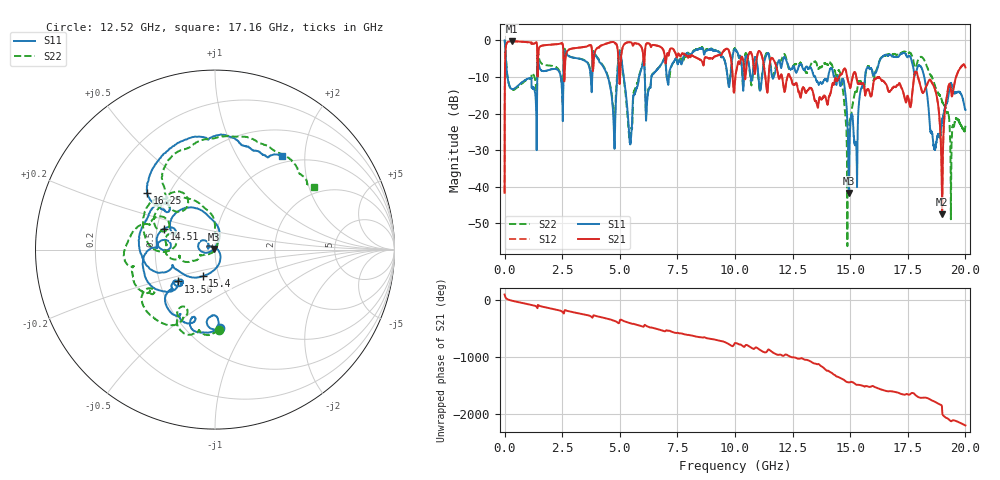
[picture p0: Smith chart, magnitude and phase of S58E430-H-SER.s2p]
!{S58E430}
!Johanson Technology Inc.
!www.johansontechnology.com
!Test Board Conditions:
!Substrate Type  RO4350B
!Substrate Thickness  60 mil
!Substrate Dk  3.66
!TL Type: GCPW
!TL Trace Width  115 mil
!TL Gap  52 mil
!Electrode orientation  Horizontal
!DUT TOPOLOGY	SERIES
!Mounting Pad LxW  55x428 mil
! Created Wed Apr 14 11:48:31 2021
# mhz S ma R 50
! 2 Port Network Data from SP1.SP block
! freq  magS11  angS11  magS21  angS21  magS12  angS12  magS22  angS22
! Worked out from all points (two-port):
!   20001 points, 300 kHz to 20 GHz, reference 50 ohm
!   highest |S21| = -0.24 dB at 309.3 MHz (marker M1); lowest = -47.5 dB at 18.99 GHz (marker M2)
!   |S21| within 3 dB of the highest: 35.1 MHz to 1.418 GHz (1.383 GHz wide, 190 % of centre); 2.697 GHz to 3.796 GHz (1.099 GHz wide, 33.8 % of centre)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
!   lowest |S11| = -41.6 dB at 14.94 GHz (marker M3), VSWR 1.02, Z = 49.3 + j0.339 ohm
!   |S11| at or under -10 dB: 125.9 MHz to 1.416 GHz (1.29 GHz wide, 167 % of centre); 14.5 GHz to 15.65 GHz (1.149 GHz wide, 7.62 % of centre); 18.21 GHz to end of sweep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
!   |S22| runs from -56.2 to 0.0 dB; largest |S21 - S12| = 0.01
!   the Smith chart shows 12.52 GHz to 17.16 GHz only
!   S11 on the Smith chart (normalised r, x): 12.52 GHz: 0.72, -0.77; 13.56 GHz: 0.62, -0.24; 14.51 GHz: 0.54, +0.14; 15.4 GHz: 0.84, -0.25; 16.25 GHz: 0.38, +0.32; 17.16 GHz: 0.88, +1.57
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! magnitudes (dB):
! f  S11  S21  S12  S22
! 300 kHz  0.0  -41.6  -41.6  0.0
! 107.3 MHz  -9.1  -0.6  -0.6  -9.0
! 309.3 MHz  -13.3  -0.2  -0.2  -13.5
! 3.334 GHz  -5.1  -1.9  -1.9  -5.1
! 4.743 GHz  -24.5  -0.5  -0.4  -20.9
! 5.028 GHz  -3.4  -7.2  -7.2  -3.3
! 5.444 GHz  -28.3  -0.5  -0.5  -26.2
! 6.667 GHz  -7.6  -1.5  -1.5  -7.6
! 10 GHz  -2.4  -11.1  -11.1  -2.3
! 12.52 GHz  -7.2  -12.0  -11.9  -6.9
! 13.33 GHz  -8.0  -13.3  -13.2  -6.2
! 13.56 GHz  -11.3  -17.5  -17.6  -6.9
! 14.51 GHz  -10.2  -10.2  -10.1  -8.2
! 14.94 GHz  -41.6  -11.8  -11.7  -24.0
! 15.4 GHz  -15.7  -11.8  -11.8  -11.3
! 16.25 GHz  -6.2  -10.0  -10.0  -6.1
! 16.67 GHz  -4.1  -13.9  -14.0  -3.8
! 17.16 GHz  -3.8  -12.0  -12.0  -3.7
! 18.12 GHz  -7.8  -14.0  -14.0  -4.6
! 18.54 GHz  -25.1  -11.5  -11.5  -9.9
! 18.99 GHz  -21.8  -47.5  -45.7  -16.7
! 20 GHz  -18.9  -7.4  -7.3  -23.3
